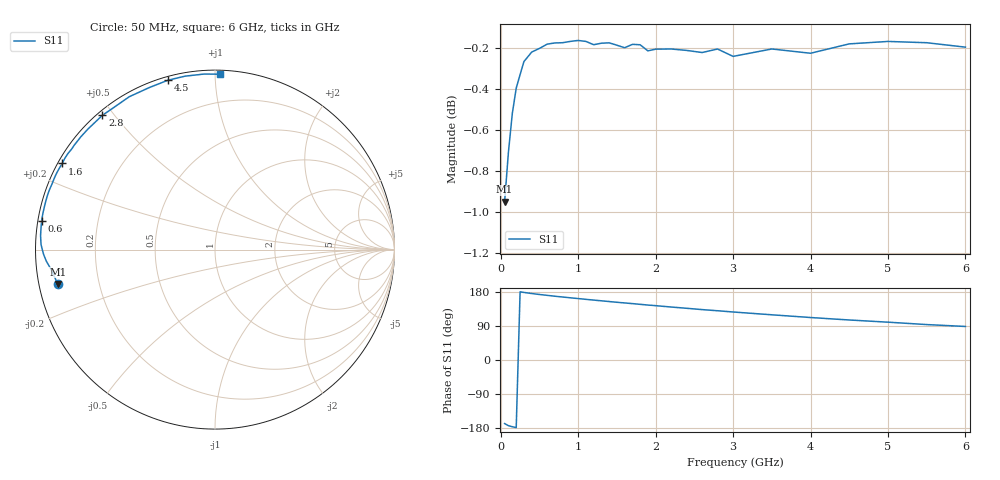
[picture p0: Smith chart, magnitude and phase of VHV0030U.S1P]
! Infineon Technologies  Discrete & RF Semiconductors
! BB 814
! Si Tuning Diode in SOT23
! VR =
! S-Parameters:  July  1999
# GHz  S  MA  R  50
!  f  S11
! GHz  MAG  ANG
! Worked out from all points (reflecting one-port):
!   34 points, 50 MHz to 6 GHz, reference 50 ohm
!   lowest |S11| = -0.9 dB at 50 MHz (marker M1), VSWR 18.32, Z = 2.76 - j5.37 ohm
!   phase of S11 starts at -168 deg and turns -104 deg over the sweep
!   S11 on the Smith chart (normalised r, x): 50 MHz: 0.06, -0.11; 600 MHz: 0.01, +0.08; 1.6 GHz: 0.01, +0.26; 2.8 GHz: 0.01, +0.47; 4.5 GHz: 0.02, +0.76; 6 GHz: 0.02, +1.03
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0.05  0.8965 -167.7
0.1  0.9221 -173.4
0.15  0.942 -176.1
0.2  0.9554 -178.4
0.3  0.9697 178.3
0.4  0.9749 175.4
0.6  0.9792 170.6
0.7  0.9798 168.3
0.8  0.98 166.2
1  0.9812 162.1
1.2  0.9789 158.1
1.4  0.9799 154.3
1.5  0.9786 152.3
1.6  0.9772 150.6
1.7  0.9791 148.8
1.9  0.9755 145.0
2  0.9764 143.4
2.2  0.9765 139.8
2.4  0.9758 136.5
2.6  0.9746 133.0
2.8  0.9765 130.0
3  0.9725 126.7
3.5  0.9765 119.3
4  0.9742 112.1
4.5  0.9793 105.6
5  0.9807 99.8
5.5  0.98 93.5
6  0.9775 88.5
